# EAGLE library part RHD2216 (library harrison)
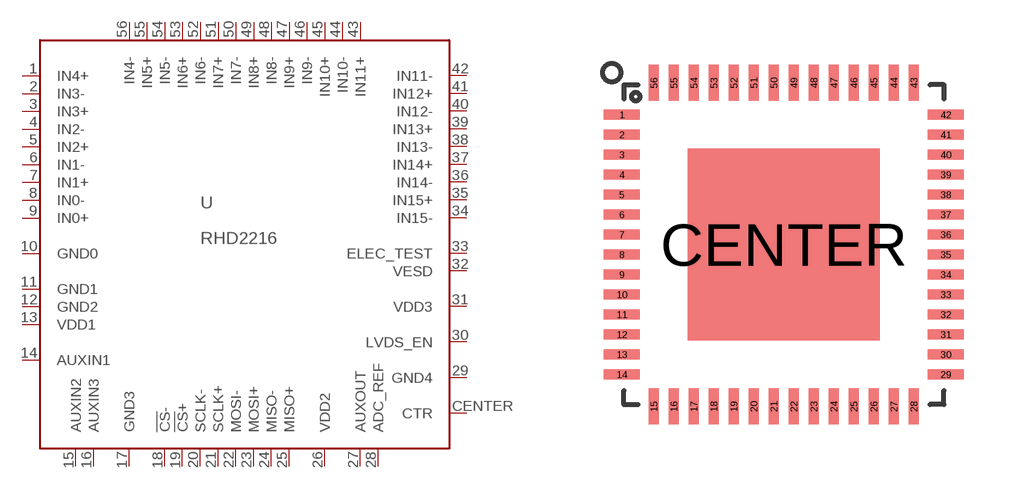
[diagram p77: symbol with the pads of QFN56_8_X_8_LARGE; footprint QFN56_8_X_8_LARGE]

Designator prefix U

## RHD2216_QFN  [QFN56_8_X_8_LARGE]
1  IN4+  in
2  IN3-  in
3  IN3+  in
4  IN2-  in
5  IN2+  in
6  IN1-  in
7  IN1+  in
8  IN0-  in
9  IN0+  in
10  GND0  in
11  GND1  pwr
12  GND2  pwr
13  VDD1  pwr
14  AUXIN1  in
15  AUXIN2  in
16  AUXIN3  in
17  GND3  pwr
18  !CS!-  in
19  !CS!+  in
20  SCLK-  in
21  SCLK+  in
22  MOSI-  in
23  MOSI+  in
24  MISO-  out
25  MISO+  out
26  VDD2  pwr
27  AUXOUT  hiz
28  ADC_REF  pas
29  GND4  pwr
30  LVDS_EN  in
31  VDD3  pwr
32  VESD  pwr
33  ELEC_TEST  in
34  IN15-  in
35  IN15+  in
36  IN14-  in
37  IN14+  in
38  IN13-  in
39  IN13+  in
40  IN12-  in
41  IN12+  in
42  IN11-  in
43  IN11+  in
44  IN10-  in
45  IN10+  in
46  IN9-  in
47  IN9+  in
48  IN8-  in
49  IN8+  in
50  IN7-  in
51  IN7+  in
52  IN6-  in
53  IN6+  in
54  IN5-  in
55  IN5+  in
56  IN4-  in
CENTER  CTR  pwr

## Footprint QFN56_8_X_8_LARGE (pad centres in mm)
smd 0.9 x 0.25: 1 -4.05,3.25; 2 -4.05,2.75; 3 -4.05,2.25; 4 -4.05,1.75; 5 -4.05,1.25; 6 -4.05,0.75; 7 -4.05,0.25; 8 -4.05,-0.25; 9 -4.05,-0.75; 10 -4.05,-1.25; 11 -4.05,-1.75; 12 -4.05,-2.25; 13 -4.05,-2.75; 14 -4.05,-3.25; 29 4.05,-3.25; 30 4.05,-2.75; 31 4.05,-2.25; 32 4.05,-1.75; 33 4.05,-1.25; 34 4.05,-0.75; 35 4.05,-0.25; 36 4.05,0.25; 37 4.05,0.75; 38 4.05,1.25; 39 4.05,1.75; 40 4.05,2.25; 41 4.05,2.75; 42 4.05,3.25
smd 0.25 x 0.9: 15 -3.25,-4.05; 16 -2.75,-4.05; 17 -2.25,-4.05; 18 -1.75,-4.05; 19 -1.25,-4.05; 20 -0.75,-4.05; 21 -0.25,-4.05; 22 0.25,-4.05; 23 0.75,-4.05; 24 1.25,-4.05; 25 1.75,-4.05; 26 2.25,-4.05; 27 2.75,-4.05; 28 3.25,-4.05; 43 3.25,4.05; 44 2.75,4.05; 45 2.25,4.05; 46 1.75,4.05; 47 1.25,4.05; 48 0.75,4.05; 49 0.25,4.05; 50 -0.25,4.05; 51 -0.75,4.05; 52 -1.25,4.05; 53 -1.75,4.05; 54 -2.25,4.05; 55 -2.75,4.05; 56 -3.25,4.05
smd 4.8 x 4.8: CENTER 0,0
